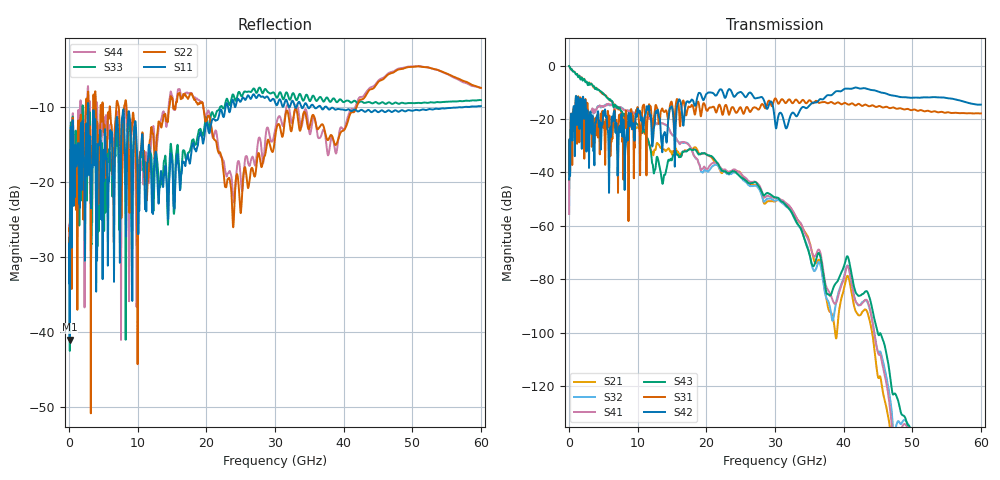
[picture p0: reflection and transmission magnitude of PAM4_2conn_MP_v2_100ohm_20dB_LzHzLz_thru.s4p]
! Info: Touchstone file created by Circ.  Input file=FAB50GbE_2conn_Midplane_Examax_Topo2_v2_100ohm_20dB_LzHzLz.circ
# Hz S RI R 50
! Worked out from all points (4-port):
!   6000 points, 10 MHz to 60 GHz, reference 50 ohm
!   strongest paths, dB at 10 MHz, 15.01 GHz, 30.01 GHz, 45.01 GHz, 60 GHz:
!     S42: -42.6, -15.7, -21.2, -9.7, -14.6
!     S31: -42.7, -14.3, -12.3, -15.2, -17.9
!     S43: -0.2, -35.0, -49.3, -100.4, -154.8
!     S41: -55.6, -25.9, -49.5, -107.6, -162.9
!     S32: -55.6, -25.8, -50.6, -107.2, -160.3
!     S21: -0.2, -33.4, -50.9, -116.6, -168.2
!   lowest |S11| = -41.0 dB at 100 MHz (marker M1), VSWR 1.02, Z = 50.1 - j0.883 ohm
!   |S11| at or under -10 dB: start of sweep to 2.747 GHz; 2.815 GHz to 22.79 GHz (19.98 GHz wide, 156 % of centre); 37.55 GHz to 57.42 GHz (19.87 GHz wide, 41.8 % of centre)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
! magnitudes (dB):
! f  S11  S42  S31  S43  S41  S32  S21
! 10 MHz  -33.5  -42.6  -42.7  -0.2  -55.6  -55.6  -0.2
! 100 MHz  -41.0  -28.2  -28.0  -0.6  -35.3  -35.3  -0.6
! 1.43 GHz  -19.5  -14.3  -14.7  -4.0  -20.1  -20.0  -3.9
! 10.26 GHz  -22.9  -17.1  -23.6  -23.5  -17.8  -17.8  -24.0
! 31.97 GHz  -9.9  -21.2  -12.8  -53.3  -52.2  -53.5  -52.3
! 37.27 GHz  -10.0  -12.0  -13.6  -81.9  -80.7  -85.0  -84.3
! 60 GHz  -9.9  -14.6  -17.9  -154.8  -162.9  -160.3  -168.2
